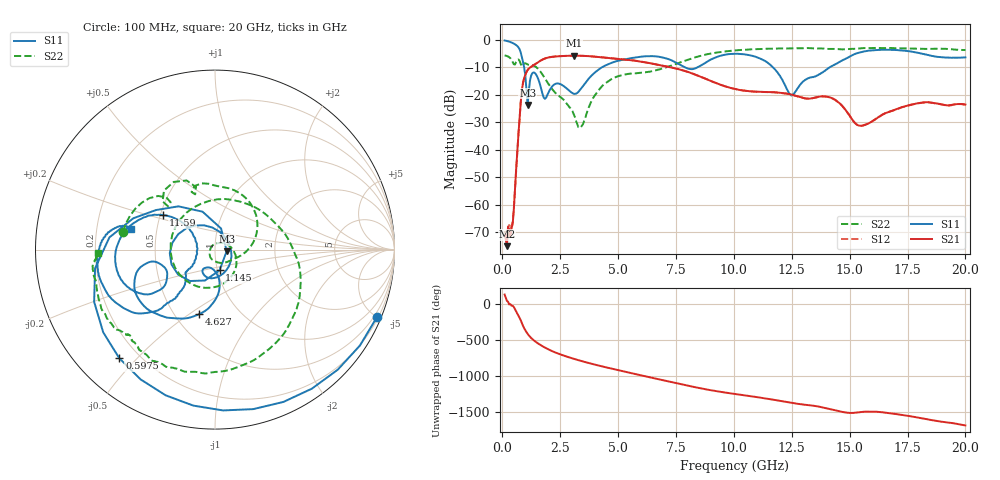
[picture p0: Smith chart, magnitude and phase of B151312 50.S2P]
!  2-Port S-parameters saved by WinCal
! VAR MeasName=S-Parameters (CALIBRATED_DATA) read from VNA (N5244A)
! VAR MeasDate=12/8/2015 5:47:44 PM
! VAR NAME=B151312 50
! VAR FILENAME=B151312 50.S2P
! VAR DATE=12/8/2015 5:47:44 PM
! VAR PHYS_PORTS=1,2
# Hz S DB R 50
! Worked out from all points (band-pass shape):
!   401 points, 100 MHz to 20 GHz, reference 50 ohm
!   highest |S21| = -5.73 dB at 3.085 GHz (marker M1); lowest = -75.0 dB at 199.5 MHz (marker M2)
!   |S21| within 3 dB of the highest: 1.434 GHz to 6.524 GHz (5.09 GHz wide, 128 % of centre)
!   lowest |S11| = -23.6 dB at 1.095 GHz (marker M3), VSWR 1.14, Z = 57 - j0.971 ohm
!   |S11| at or under -10 dB: 945.2 MHz to 4.294 GHz (3.348 GHz wide, 128 % of centre); 7.898 GHz to 8.42 GHz (521.8 MHz wide, 6.4 % of centre); 11.7 GHz to 14.13 GHz (2.438 GHz wide, 18.9 % of centre)
!   |S22| runs from -31.9 to -2.9 dB; largest |S21 - S12| = 0.0018
!   S11 on the Smith chart (normalised r, x): 100 MHz: 0.29, -4.99; 597.5 MHz: 0.13, -0.45; 1.145 GHz: 1.02, -0.24; 4.627 GHz: 0.66, -0.55; 11.59 GHz: 0.52, +0.22; 20 GHz: 0.35, +0.10
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1e8  -0.20 -22.6  -70.84 137.4  -69.48 140.8  -5.64 169.3
1.995e8  -0.38 -44.4  -74.98 49.0  -73.08 56.3  -5.85 158.4
4.4825e8  -1.13 -97.9  -67.01 -19.6  -66.16 -11.6  -8.00 133.0
5.975e8  -1.86 -131.3  -47.10 -100.9  -47.11 -101.2  -8.02 137.4
8.4625e8  -6.24 159.0  -18.29 98.0  -18.30 97.9  -9.70 109.7
1.095e9  -23.65 -7.4  -10.94 -53.1  -10.93 -53.2  -8.91 90.9
1.14475e9  -18.53 -77.8  -10.42 -74.3  -10.42 -74.3  -9.04 86.8
1.54275e9  -14.00 143.6  -8.10 173.3  -8.10 173.2  -10.47 40.2
2.04025e9  -18.33 -50.4  -6.30 82.0  -6.30 82.0  -16.55 -12.6
3.085e9  -19.58 -109.2  -5.73 -42.0  -5.73 -42.0  -27.02 -129.3
3.43325e9  -17.35 -85.8  -5.78 -74.9  -5.77 -74.9  -31.22 117.2
4.62725e9  -8.64 -103.7  -6.61 -172.8  -6.59 -172.8  -14.72 -66.0
5.72175e9  -6.42 -130.0  -7.54 106.2  -7.53 106.2  -12.14 -176.7
6.7665e9  -6.12 -155.3  -9.11 30.7  -9.11 30.6  -10.77 74.6
8.10975e9  -10.60 -158.7  -11.90 -65.1  -11.89 -65.1  -6.97 -3.8
1.005e10  -5.04 -170.6  -17.84 -175.0  -17.82 -175.3  -3.83 -66.9
1.159225e10  -9.19 146.6  -18.98 111.2  -19.02 111.0  -3.21 -97.0
1.248775e10  -20.24 177.3  -19.90 61.2  -19.92 61.1  -3.06 -111.2
1.338325e10  -13.51 -141.3  -21.22 23.4  -21.22 23.3  -3.07 -122.3
1.5423e10  -4.60 -144.8  -31.16 -69.9  -31.16 -69.7  -3.10 -140.2
1.67165e10  -3.61 -172.3  -26.13 -83.8  -26.07 -84.4  -2.93 -152.3
2e10  -6.35 166.5  -23.49 104.7  -23.59 104.2  -3.69 -178.2
